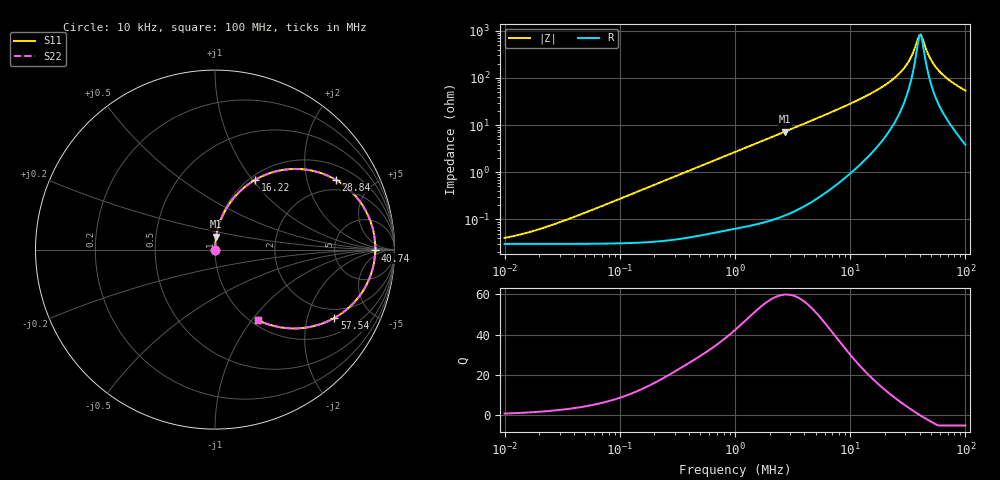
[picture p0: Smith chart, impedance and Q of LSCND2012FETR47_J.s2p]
! LSCND2012FETR47_J  S-PARAMETER MODEL  ( Standard Model )
! Model Generated by TAIYO YUDEN Corporation (http://www.ty-top.com)
! Version 1.0
! TAIYO YUDEN Control No. 241216
! Copyright(c) 2025 TAIYO YUDEN CO.,LTD. All Rights Reserved.
! Product Description (link to TY-COMPAS)
! https://ds.yuden.co.jp/TYCOMPAS/or/detail?pn=LSCND2012FETR47MJ&u=M
! Products Name : Inductors
! Characteristics :
!  Inductance : 0.47 [uH] , SRF(min) : - [Hz] , DC Resistance(max) : 34 [mOhm]
!  Rated Current : Saturation  4.5 [A] (dL = 30 [%]), Temp Rise  3.7 [A] (dT = 40 [degC])
!  Case Size : 2.0 x 1.2 / 0.079 x 0.047 [mm/inch] , Thickness : 0.65 / 0.026 [mm/inch]
!  (Conditions: Temperature = 25 [degC] , DC Bias Current = 0 [A])
! External Node Assignments :
!  1  o---GGG---o  2
! GND o---------o GND
! Frequency Range : 10kHz  -  100MHz  [ 402 STEP ]
# MHz S RI R 50
! Freq[MHz].  S11 Real  S11 Imag  S21 Real  S21 Imag  S12 Real  S12 Imag  S22 Real  S22 Imag
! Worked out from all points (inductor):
!   401 points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, 10 kHz to 100 MHz, reference 50 ohm
!   read as one part in series: L = 433 nH near 33.88 kHz
!   highest Q = 59.9 at 2.692 MHz (marker M1), where L = 426 nH
!   self-resonance near 40.6 MHz
!   S11 on the Smith chart (normalised r, x): 10 kHz: 1.00, +0.00; 16.22 MHz: 1.06, +1.03; 28.84 MHz: 1.53, +3.01; 40.74 MHz: 18, -1; 57.54 MHz: 1.60, -2.96; 100 MHz: 1.08, -1.08
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0.01  0.000303 0.000272  0.9997 -0.000272  0.9997 -0.000272  0.000303 0.000272
0.019498  0.000303 0.00053  0.9997 -0.00053  0.9997 -0.00053  0.000303 0.00053
0.046774  0.000306 0.00127  0.9997 -0.00127  0.9997 -0.00127  0.000306 0.00127
0.218776  0.000379 0.00594  0.9996 -0.00594  0.9996 -0.00594  0.000379 0.00594
1  0.00135 0.0268  0.9986 -0.0268  0.9986 -0.0268  0.00135 0.0268
2.691535  0.00636 0.0716  0.9936 -0.0716  0.9936 -0.0716  0.00636 0.0716
4.677351  0.018 0.1238  0.982 -0.1238  0.982 -0.1238  0.018 0.1238
10  0.0818 0.2579  0.9182 -0.2579  0.9182 -0.2579  0.0818 0.2579
16.2181  0.2218 0.3876  0.7782 -0.3876  0.7782 -0.3876  0.2218 0.3876
21.87762  0.4095 0.4478  0.5905 -0.4478  0.5905 -0.4478  0.4095 0.4478
25.11886  0.5334 0.4414  0.4666 -0.4414  0.4666 -0.4414  0.5334 0.4414
28.84032  0.6731 0.3889  0.3269 -0.3889  0.3269 -0.3889  0.6731 0.3889
33.11311  0.8039 0.2728  0.1961 -0.2728  0.1961 -0.2728  0.8039 0.2728
35.48134  0.853 0.1903  0.147 -0.1903  0.147 -0.1903  0.853 0.1903
38.90451  0.8895 0.0626  0.1105 -0.0626  0.1105 -0.0626  0.8895 0.0626
40.73803  0.893 -0.00486  0.107 0.00486  0.107 0.00486  0.893 -0.00486
42.65795  0.8862 -0.0718  0.1138 0.0718  0.1138 0.0718  0.8862 -0.0718
48.97788  0.8118 -0.2494  0.1882 0.2494  0.1882 0.2494  0.8118 -0.2494
52.48075  0.753 -0.3168  0.247 0.3168  0.247 0.3168  0.753 -0.3168
57.54399  0.6649 -0.3812  0.3351 0.3812  0.3351 0.3812  0.6649 -0.3812
72.4436  0.4518 -0.439  0.5482 0.439  0.5482 0.439  0.4518 -0.439
100  0.2404 -0.3933  0.7596 0.3933  0.7596 0.3933  0.2404 -0.3933
